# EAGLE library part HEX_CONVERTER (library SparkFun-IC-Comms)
74HC4050 Hex Buffer 74HC4050 Hex Buffer Level Shifter SMD SO016 SparkFun Products CAN-BUS Shield (DEV-13262) SparkFun MP3 Player Shield (DEV-12660) SparkFun microSD Shield (DEV-12761) SparkFun USB Host Shield (DEV-09947)
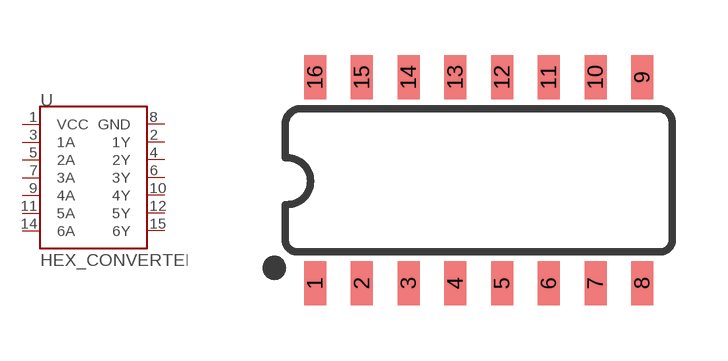
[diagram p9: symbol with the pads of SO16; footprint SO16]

Designator prefix U

## HEX_CONVERTER (PROD_ID: IC-09604; VALUE: 74HC4050)  [SO16]
1  VCC
2  1Y
3  1A
4  2Y
5  2A
6  3Y
7  3A
8  GND
9  4A
10  4Y
11  5A
12  5Y
14  6A
15  6Y

## Footprint SO16 (pad centres in mm)
SOIC-16 Specifications: Pin count: 16 Width:0.15" Example device(s): HEX_CONVERTER
smd 0.6 x 1.2: 1 -4.445,-2.8; 2 -3.175,-2.8; 3 -1.905,-2.8; 4 -0.635,-2.8; 5 0.635,-2.8; 6 1.905,-2.8; 7 3.175,-2.8; 8 4.445,-2.8; 9 4.445,2.8; 10 3.175,2.8; 11 1.905,2.8; 12 0.635,2.8; 13 -0.635,2.8; 14 -1.905,2.8; 15 -3.175,2.8; 16 -4.445,2.8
